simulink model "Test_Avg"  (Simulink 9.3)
settings: Solver=VariableStepAuto  StartTime=0.0  StopTime=0.5  RelTol=1e-3
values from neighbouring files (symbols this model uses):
  Tstep = 0.000050    (= 5e-05)    [TestOrthOsc_init.m]    (also in Test_PIDctrl_init.m = 0.0001)
libraries: libVishia_CtrlSfn x7, libVishia_Conv x1

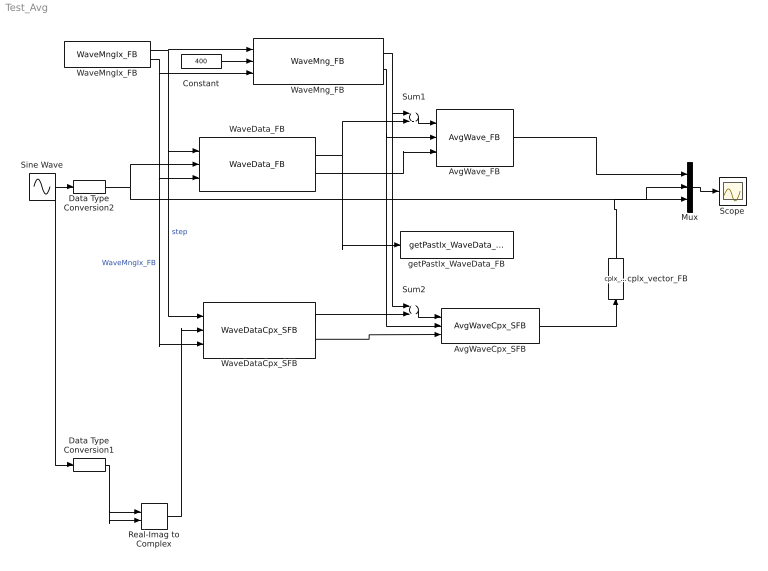
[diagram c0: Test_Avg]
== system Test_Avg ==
  AvgWaveCpx_SFB : libVishia_CtrlSfn/AvgWaveCpx_SFB  SystemSampleTime=-1
  AvgWave_FB : libVishia_CtrlSfn/AvgWave_FB  identObj=1
  Constant : Constant  Value=400  OutDataTypeStr=single
  Data Type Conversion1 : DataTypeConversion  OutDataTypeStr=single
  Data Type Conversion2 : DataTypeConversion  OutDataTypeStr=single
  Mux : Mux  Inputs=3
  Real-Imag to Complex : RealImagToComplex
  Scope : Scope
  Sine Wave : Sin  Amplitude=4  Frequency=10.02*pi  SampleTime=Tstep
  Sum1 : Sum
  Sum2 : Sum
  WaveDataCpx_SFB : libVishia_CtrlSfn/WaveDataCpx_SFB  sizeData=1024
  WaveData_FB : libVishia_CtrlSfn/WaveData_FB  identObj=1  size=1024
  WaveMngIx_FB : libVishia_CtrlSfn/WaveMngIx_FB  identObj=1  size=1024  Tstep=Tstep
  WaveMng_FB : libVishia_CtrlSfn/WaveMng_FB  identObj=1
  cplx_vector_FB : libVishia_Conv/cplx_vector_FB  SystemSampleTime=-1
  getPastIx_WaveData_FB : libVishia_CtrlSfn/getPastIx_WaveData_FB  Commented=on  ixPast=25
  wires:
  Constant/1 -> WaveMng_FB/2
  WaveData_FB/1 -> Sum1/2, getPastIx_WaveData_FB/1
  Sum1/1 -> AvgWave_FB/1
  WaveData_FB/2 -> AvgWave_FB/3
  Mux/1 -> Scope/1
  AvgWave_FB/1 -> Mux/1
  Data Type Conversion2/1 -> WaveData_FB/2, Mux/2
  Data Type Conversion1/1 -> Real-Imag to Complex/2, Real-Imag to Complex/1
  Sine Wave/1 -> Data Type Conversion1/1, Data Type Conversion2/1
  Real-Imag to Complex/1 -> WaveDataCpx_SFB/2
  WaveMngIx_FB/1 -> WaveDataCpx_SFB/1, WaveData_FB/1, WaveMng_FB/1  "step"
  WaveMngIx_FB/2 -> WaveMng_FB/3, WaveDataCpx_SFB/3, WaveData_FB/3  "WaveMngIx_FB"
  WaveMng_FB/1 -> Sum2/1, Sum1/1
  WaveMng_FB/2 -> AvgWaveCpx_SFB/2, AvgWave_FB/2
  WaveDataCpx_SFB/1 -> Sum2/2
  Sum2/1 -> AvgWaveCpx_SFB/1
  WaveDataCpx_SFB/2 -> AvgWaveCpx_SFB/3
  AvgWaveCpx_SFB/1 -> cplx_vector_FB/1
  cplx_vector_FB/1 -> Mux/3
